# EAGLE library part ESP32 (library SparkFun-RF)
Espressif ESP32 WiFi-compatible SoC microcontroller. Bluetooth Low energy support (BLE, BT4.0, Bluetooth Smart) 28 GPIO pins Dual-core Tensilica LX6 microprocessor Hardware accelerated encryption (AES, SHA2, ECC, RSA-4096) 4MB Flash memory 520kB internal SRAM Datasheet SparkFun Products: SparkFun ESP32 Thing
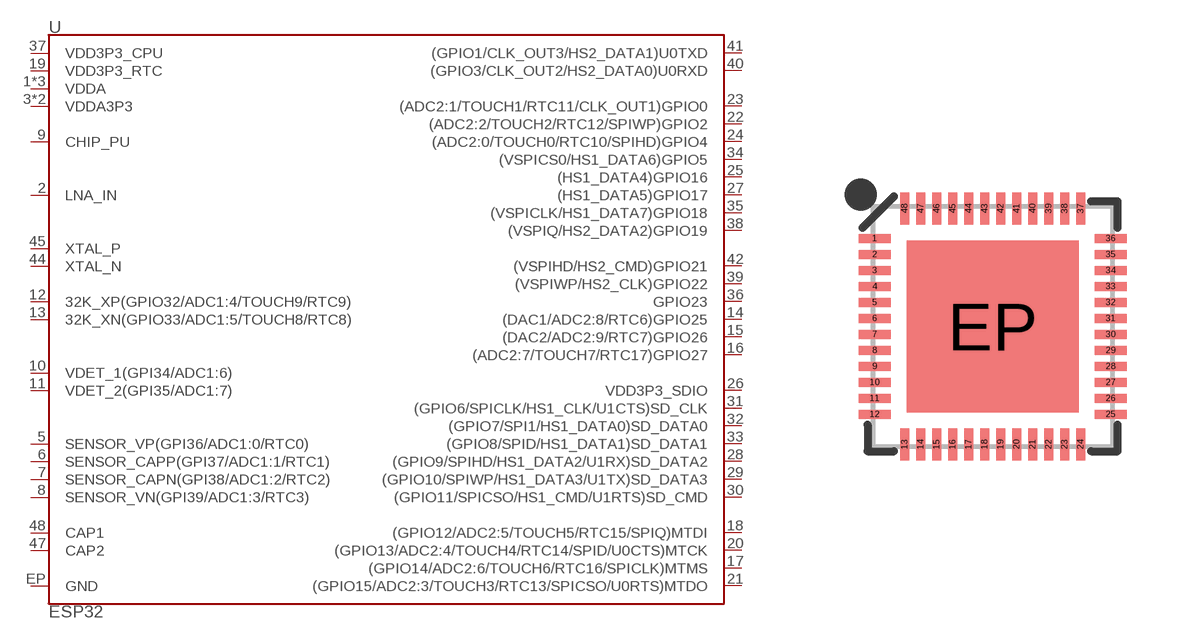
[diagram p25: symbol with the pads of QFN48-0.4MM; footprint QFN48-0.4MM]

Designator prefix U

## ESP32 (PROD_ID: IC-13338)  [QFN48-0.4MM]
1  VDDA
2  LNA_IN
3  VDDA3P3
4  VDDA3P3
5  SENSOR_VP(GPI36/ADC1:0/RTC0)
6  SENSOR_CAPP(GPI37/ADC1:1/RTC1)
7  SENSOR_CAPN(GPI38/ADC1:2/RTC2)
8  SENSOR_VN(GPI39/ADC1:3/RTC3)
9  CHIP_PU
10  VDET_1(GPI34/ADC1:6)
11  VDET_2(GPI35/ADC1:7)
12  32K_XP(GPIO32/ADC1:4/TOUCH9/RTC9)
13  32K_XN(GPIO33/ADC1:5/TOUCH8/RTC8)
14  (DAC1/ADC2:8/RTC6)GPIO25
15  (DAC2/ADC2:9/RTC7)GPIO26
16  (ADC2:7/TOUCH7/RTC17)GPIO27
17  (GPIO14/ADC2:6/TOUCH6/RTC16/SPICLK)MTMS
18  (GPIO12/ADC2:5/TOUCH5/RTC15/SPIQ)MTDI
19  VDD3P3_RTC
20  (GPIO13/ADC2:4/TOUCH4/RTC14/SPID/U0CTS)MTCK
21  (GPIO15/ADC2:3/TOUCH3/RTC13/SPICSO/U0RTS)MTDO
22  (ADC2:2/TOUCH2/RTC12/SPIWP)GPIO2
23  (ADC2:1/TOUCH1/RTC11/CLK_OUT1)GPIO0
24  (ADC2:0/TOUCH0/RTC10/SPIHD)GPIO4
25  (HS1_DATA4)GPIO16
26  VDD3P3_SDIO
27  (HS1_DATA5)GPIO17
28  (GPIO9/SPIHD/HS1_DATA2/U1RX)SD_DATA2
29  (GPIO10/SPIWP/HS1_DATA3/U1TX)SD_DATA3
30  (GPIO11/SPICSO/HS1_CMD/U1RTS)SD_CMD
31  (GPIO6/SPICLK/HS1_CLK/U1CTS)SD_CLK
32  (GPIO7/SPI1/HS1_DATA0)SD_DATA0
33  (GPIO8/SPID/HS1_DATA1)SD_DATA1
34  (VSPICS0/HS1_DATA6)GPIO5
35  (VSPICLK/HS1_DATA7)GPIO18
36  GPIO23
37  VDD3P3_CPU
38  (VSPIQ/HS2_DATA2)GPIO19
39  (VSPIWP/HS2_CLK)GPIO22
40  (GPIO3/CLK_OUT2/HS2_DATA0)U0RXD
41  (GPIO1/CLK_OUT3/HS2_DATA1)U0TXD
42  (VSPIHD/HS2_CMD)GPIO21
43  VDDA
44  XTAL_N
45  XTAL_P
46  VDDA
47  CAP2
48  CAP1
EP  GND

## Footprint QFN48-0.4MM (pad centres in mm)
QFN 48 Pin Specifications: Pin count: 48 Pin pitch: 0.4mm Datasheet referenced for footprint Example device(s): ESP32
smd 0.8 x 0.23: 1 -2.95,2.2; 2 -2.95,1.8; 3 -2.95,1.4; 4 -2.95,1; 5 -2.95,0.6; 6 -2.95,0.2; 7 -2.95,-0.2; 8 -2.95,-0.6; 9 -2.95,-1; 10 -2.95,-1.4; 11 -2.95,-1.8; 12 -2.95,-2.2; 25 2.95,-2.2; 26 2.95,-1.8; 27 2.95,-1.4; 28 2.95,-1; 29 2.95,-0.6; 30 2.95,-0.2; 31 2.95,0.2; 32 2.95,0.6; 33 2.95,1; 34 2.95,1.4; 35 2.95,1.8; 36 2.95,2.2
smd 0.23 x 0.8: 13 -2.2,-2.95; 14 -1.8,-2.95; 15 -1.4,-2.95; 16 -1,-2.95; 17 -0.6,-2.95; 18 -0.2,-2.95; 19 0.2,-2.95; 20 0.6,-2.95; 21 1,-2.95; 22 1.4,-2.95; 23 1.8,-2.95; 24 2.2,-2.95; 37 2.2,2.95; 38 1.8,2.95; 39 1.4,2.95; 40 1,2.95; 41 0.6,2.95; 42 0.2,2.95; 43 -0.2,2.95; 44 -0.6,2.95; 45 -1,2.95; 46 -1.4,2.95; 47 -1.8,2.95; 48 -2.2,2.95
smd 4.3 x 4.3: EP 0,0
